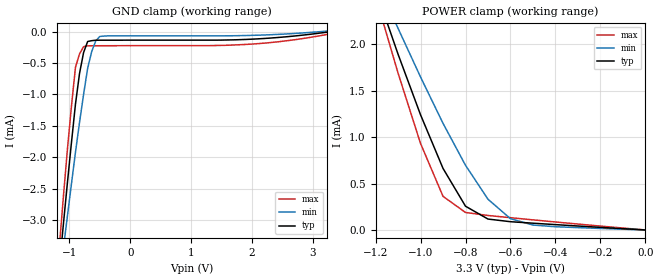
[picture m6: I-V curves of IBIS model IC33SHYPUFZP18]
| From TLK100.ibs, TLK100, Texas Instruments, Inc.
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|   Model Cell IC33SHYPUFZP18
[Model]   IC33SHYPUFZP18
Model_type   Input
Polarity   Non-Inverting
Vinl =  0.8V
Vinh =  2V
C_comp   0.8987711p   0.7775247p   0.94326p
[Model Spec]
Vinl   0.8V   0.8V   0.8V
Vinh   2V   2V   2V
[Temperature Range]   25   125   -40
[Voltage Range]   3.3   3.13   3.47
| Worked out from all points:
|   GND clamp passes 1 mA (typ) near -0.88 V on its own axis
|   POWER clamp passes 1 mA (typ) near -0.96 V on its own axis
[POWER_clamp]
|   voltage   I(typ)   I(min)   I(max)
-3.3V     17.71mA    14.37mA    20.92mA
-1.167V   2.359mA    2.531mA    2.241mA
-1.133V   2.126mA    2.352mA    1.966mA
-1.1V     1.894mA    2.172mA    1.69mA
-1.067V   1.676mA    1.997mA    1.438mA
-1V       1.241mA    1.647mA    931.9uA
-900mV    663.2uA    1.148mA    362.3uA
-800mV    255.9uA    696.2uA    188.5uA
-700mV    117.6uA    330.9uA    156.2uA
-600mV    89.11uA    121.5uA    132.2uA
-500mV    73uA       53.01uA    108.9uA
-11.55fV  95.23nA    89.73nA    222.7nA
[GND_clamp]
|   voltage   I(typ)   I(min)   I(max)
-3.3V     -26.2mA    -21.58mA   -29.28mA
-1.167V   -3.771mA   -4mA       -3.451mA
-1.1V     -3.083mA   -3.467mA   -2.648mA
-1.033V   -2.417mA   -2.944mA   -1.888mA
-900mV    -1.156mA   -1.923mA   -569uA
-833.3mV  -666.4uA   -1.446mA   -354.7uA
-766.7mV  -333.7uA   -999.9uA   -240.5uA
-700mV    -157.8uA   -585.2uA   -226.4uA
-566.7mV  -137.7uA   -148uA     -225.4uA
-500mV    -137.1uA   -77.34uA   -225.3uA
1.9V      -124.8uA   -62.39uA   -204.2uA
3.233V    -8.72uA    8.46uA     -45.2uA
